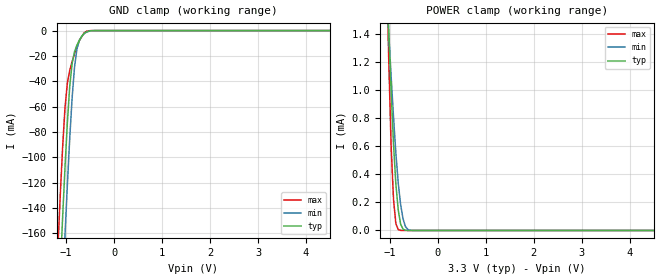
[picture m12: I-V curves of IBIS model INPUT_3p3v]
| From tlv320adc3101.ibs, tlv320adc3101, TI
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|   INPUT_3p3v
[Model]   INPUT_3p3v
Model_type   Input
Vinl = 0.99
Vinh = 2.31
|   typ   min   max
C_comp   1.022pF   1.010pF   1.056pF
[Voltage Range]   3.3   3   3.6
[Temperature Range]   27   85   -40
[Power Clamp Reference]   3.3   3   3.6
[GND Clamp Reference]   -0   -0   -0
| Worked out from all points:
|   GND clamp passes 1 mA (typ) near -0.57 V on its own axis
|   POWER clamp passes 1 mA (typ) near -0.97 V on its own axis
[GND Clamp]
|   Voltage   I(typ)   I(min)   I(max)
-3.3V     -2.298A    -2.352A    -2.242A
-1.171V   -232.3mA   -290.1mA   -171.4mA
-1.122V   -188.9mA   -246mA     -129.8mA
-1.073V   -147.1mA   -202.9mA   -91.84mA
-1.023V   -107.6mA   -161.1mA   -60.72mA
-973.5mV  -72.17mA   -121.3mA   -41.26mA
-924mV    -43.71mA   -84.61mA   -31.36mA
-874.5mV  -25.68mA   -52.82mA   -24.44mA
-825mV    -16.7mA    -28.85mA   -18.34mA
-726mV    -7.714mA   -8.012mA   -8.077mA
-577.5mV  -1.028mA   -1.218mA   -588.6uA
6.551V    0A         0A         0A
[POWER Clamp]
|   Voltage   I(typ)   I(min)   I(max)
-3.3V     25.22mA    17.7mA     43.56mA
-1.073V   1.863mA    1.718mA    1.949mA
-1.023V   1.411mA    1.401mA    1.206mA
-973.5mV  988.1uA    1.095mA    599.1uA
-924mV    614.9uA    807.3uA    219.9uA
-874.5mV  328uA      548.3uA    47.42uA
-825mV    144.1uA    335.7uA    5.833uA
-775.5mV  45.01uA    183uA      595nA
-726mV    9.583uA    83.56uA    49.23nA
-676.5mV  1.696uA    28.89uA    24.62nA
-577.5mV  36.61nA    1.816uA    0A
6.551V    0A         0A         0A
